// Digital input (DI) / output (DO) tests.
// PiXtend DIs are wired to EB 1
// PiXtend DOs are wired to AB 1
FUNCTION FC 1 : VOID
BEGIN
	// Calculate the expected EB 1 from AB 1.
	// The fake PiXtend spidev module wires DI do DO in the following way:
	// EB1 := ((AB1 & 0x3F) | (((AB1 ^ 0x03) & 0x03) << 6))
	L		AB 1
	UW		W#16#3F
	L		AB 1
	XOW		W#16#03
	UW		W#16#03
	SLW		6
	OW
	T		MB 10

	// Compare the actual EB 1 to the expected EB 1 (MB 10)
	L		EB 1
	L		MB 10
	__ASSERT==	__ACCU 1,	__ACCU 2

	// Increment the EB 1 / AB 1 test pattern by one
	L		AB 1
	+		1
	T		AB 1
END_FUNCTION


// GPIO tests
// PiXtend GPIO 0, 1 are wired to A 2.0, A 2.1
// PiXtend GPIO 2, 3 are wired to E 2.0, E 2.1
FUNCTION FC 2 : VOID
BEGIN
	// Calculate the expected E 2.0, E 2.1 from A 2.0, A 2.1
	// The fake PiXtend spidev module wires GPIO 0, 1 to GPIO 2, 3
	L		AB 2
	UW		W#16#03
	T		MB 20

	// Compare the actual EB 1 to the expected EB 1 (MB 20)
	L		EB 2
	L		MB 20
	__ASSERT==	__ACCU 1,	__ACCU 2

	// Increment the EB 2 / AB 2 test pattern by one
	L		AB 2
	+		1
	T		AB 2
END_FUNCTION


// Analog input tests
FUNCTION FC 3 : VOID
BEGIN
	// Check AI0
	// The fake PiXtend spidev module always reports 1 V
	L		EW 10
	L		2754
	__ASSERT==	__ACCU 1,	__ACCU 2

	// Check AI1
	// The fake PiXtend spidev module always reports 2 V
	L		EW 12
	L		5535
	__ASSERT==	__ACCU 1,	__ACCU 2

	// Check AI2
	// The fake PiXtend spidev module always reports 20.1 mA
	L		EW 14
	L		27663
	__ASSERT==	__ACCU 1,	__ACCU 2

	// Check AI3
	// The fake PiXtend spidev module always reports 14.1 mA
	L		EW 16
	L		17295
	__ASSERT==	__ACCU 1,	__ACCU 2
END_FUNCTION


ORGANIZATION_BLOCK OB 1
BEGIN
	// This test only works with the fake PiXtend-Spidev module

	CALL		FC 1	// Test DI/DO
	CALL		FC 2	// Test GPIOs
	CALL		FC 3	// Test analog inputs

	// If we ran 256 test cycles then exit.
	L		MW 100
	+		1
	T		MW 100
	L		256
	<I
	BEB
	CALL		SFC 46 // Exit test; Stop CPU.
END_ORGANIZATION_BLOCK


ORGANIZATION_BLOCK OB 100
BEGIN
	L		0
	T		AB 1
	T		AB 2
	T		MW 100
END_ORGANIZATION_BLOCK
